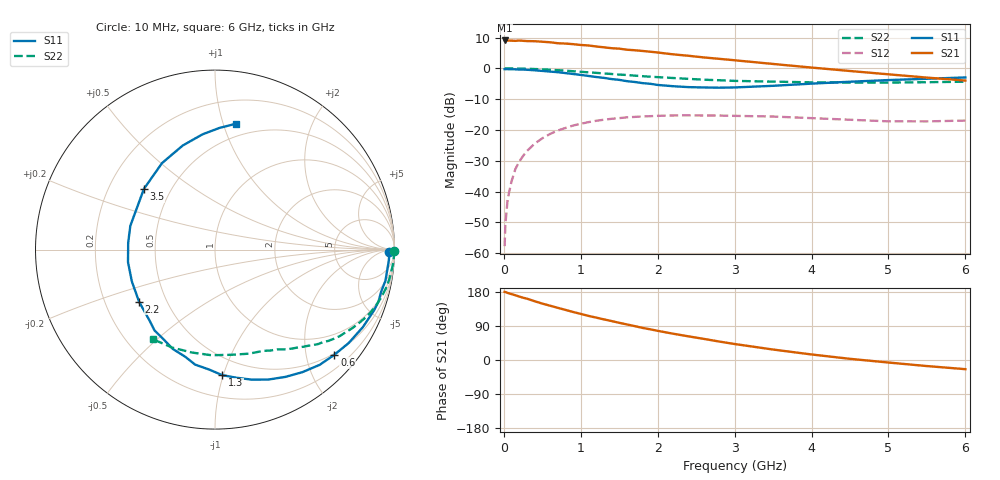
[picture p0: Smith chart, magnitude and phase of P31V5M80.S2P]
! SIEMENS Small Signal Semiconductors
! BFP181
! Si NPN RF Bipolar Junction Transistor in SOT143
! VCE = 1.5 V  IC = 0.8 mA
! Common Emitter S-Parameters:  March  1996
# GHz  S  MA  R  50
!  f  S11  S21  S12  S22
! GHz  MAG  ANG  MAG  ANG  MAG  ANG  MAG  ANG
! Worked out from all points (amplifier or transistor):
!   36 points, 10 MHz to 6 GHz, reference 50 ohm
!   highest |S21| = 9.1 dB at 10 MHz (marker M1)
!   |S21| within 3 dB of that: start of sweep to 1.598 GHz
!   unconditionally stable (mu >= 1): 3.258 GHz to end of sweep
!   at 250 MHz: K = 0.09, MSG = 18.7 dB, |S12| = -28.5 dB
!   at 1.4 GHz: K = 0.48, MSG = 11.5 dB, |S12| = -16.4 dB
!   at 6 GHz: K = 1.36, MAG = 2.9 dB, |S12| = -16.9 dB
!   S11 on the Smith chart (normalised r, x): 10 MHz: 55, -26; 600 MHz: 0.47, -2.57; 1.3 GHz: 0.36, -0.99; 2.2 GHz: 0.35, -0.27; 3.5 GHz: 0.35, +0.33; 6 GHz: 0.39, +1.11
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0.01  0.9706 -0.8  2.837 179.7  0.0013 87.1  0.9997 -0.3
0.02  0.9703 -1.5  2.813 179.4  0.0029 85.2  0.9985 -0.7
0.05  0.9707 -3.3  2.83 177.0  0.0076 90.9  0.9977 -1.7
0.1  0.9663 -7.0  2.814 173.9  0.0147 86.0  0.9969 -3.3
0.15  0.9653 -10.4  2.795 170.8  0.0232 82.3  0.9943 -4.9
0.2  0.955 -14.2  2.827 167.5  0.0306 80.7  0.9911 -6.6
0.3  0.9486 -20.9  2.772 161.9  0.0455 76.1  0.9843 -9.9
0.5  0.9088 -34.9  2.706 148.8  0.0733 66.5  0.9629 -16.2
0.6  0.8864 -41.4  2.652 143.3  0.0861 62.1  0.9489 -19.3
0.9  0.8102 -61.1  2.472 126.7  0.118 50.0  0.8981 -27.4
1.1  0.7531 -74.2  2.352 116.4  0.134 42.6  0.8617 -32.3
1.3  0.7007 -86.7  2.196 107.2  0.1467 35.7  0.8274 -36.9
1.5  0.6502 -99.8  2.088 98.1  0.1557 30.1  0.7922 -40.6
1.8  0.5764 -119.8  1.916 84.8  0.1657 22.7  0.7467 -45.8
2.2  0.513 -145.6  1.689 69.4  0.1721 13.9  0.6975 -52.3
2.4  0.496 -159.1  1.601 62.4  0.1728 9.9  0.6755 -55.4
2.8  0.4852 175.5  1.428 48.7  0.1715 3.8  0.6416 -61.2
3.5  0.5208 139.5  1.179 27.6  0.1652 -4.4  0.6095 -72.1
4  0.5652 121.5  1.03 14.6  0.1557 -8.1  0.5926 -81.5
4.5  0.6068 107.3  0.906 3.1  0.1465 -10.2  0.5889 -91.9
5.5  0.6779 88.0  0.708 -16.0  0.1378 -6.7  0.5958 -113.6
6  0.7119 80.4  0.634 -24.2  0.1421 -4.6  0.6076 -124.8
